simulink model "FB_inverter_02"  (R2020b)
settings: Solver=ode23t  StartTime=0.0  StopTime=0.001  MaxStep=1e-5  RelTol=1e-5
libraries: powerlib x7, simulink x2

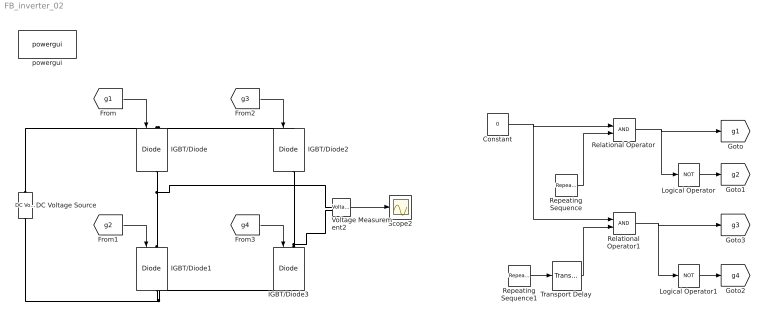
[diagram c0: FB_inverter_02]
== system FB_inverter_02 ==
  Constant : Constant  Value=0
  DC Voltage Source : powerlib/Electrical Sources/DC Voltage Source  Amplitude=400  Measurements=None
  IGBT/Diode{,1..3} (4 alike) : powerlib/Power Electronics/IGBT//Diode  Ron=1e-3  Rs=1e5  Cs=inf  Measurements=on
  Logical Operator : Logic  Operator=NOT  AllPortsSameDT=off  OutDataTypeStr=boolean
  Logical Operator1 : Logic  Operator=NOT  AllPortsSameDT=off  OutDataTypeStr=boolean
  Relational Operator : RelationalOperator  OutDataTypeStr=boolean  RndMeth=Simplest
  Relational Operator1 : RelationalOperator  OutDataTypeStr=boolean  RndMeth=Simplest
  Repeating Sequence : simulink/Sources/Repeating Sequence  rep_seq_t=[0 0.0001 0.0002]  rep_seq_y=[-400 400 -400]
  Repeating Sequence1 : simulink/Sources/Repeating Sequence  rep_seq_t=[0 0.0001 0.0002]  rep_seq_y=[-400 400 -400]
  Scope2 : Scope
  Transport Delay : TransportDelay  DelayTime=0.00001
  Voltage Measurement2 : powerlib/Measurements/Voltage Measurement  PhasorSimulation=off  OutputType=Complex  PSBequivalent=0
  powergui : powerlib/powergui  Priority=1  SimulationMode=Continuous  SampleTime=50e-6  frequency=60  Iterations=50  frequencyindice=0  Pbase=100e6  ErrMax=1e-4  UnitsV=kV  UnitsW=MW  buscounter=0  FunctionMessages=on  echomessages=on  EnableUseOfTLC=off  CurrentSourceSwitches=on  DisableSnubberDevices=on  DisableRonSwitches=on  DisableVfSwitches=on  DisplayEquations=off  AutomaticDiscreteSolvers=off  SolverType=Tustin/Backward Euler (TBE)  Interpol=off  ExternalGateDelay=off  methode=off  Ts=100  x0status=blocks  SPID=on  SwTol=0  HookPort=off  NonlinearTolerance=1e-4  nMaxIteration=100  ContinueOnMaxIteration=off  RestoreLinks=warning  ResistiveCurrentMeasurement=off  Frange=[0:2:500]  Ylog=off  Xlog=on  ShowGrid=off  save=off  variable=ZData  structure=0  ZoomFFT=off  StartTime=0.0  cycles=1  DisplayStyle=1  fundamental=60  FreqAxis=off  MaxFrequency=1000  frequencyindicesteady=1  RmsSteady=1  display=off
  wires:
  [g4] -> IGBT/Diode3/1
  [g2] -> IGBT/Diode1/1
  [g1] -> IGBT/Diode/1
  [g3] -> IGBT/Diode2/1
  Repeating Sequence/1 -> Relational Operator/2
  Constant/1 -> Relational Operator1/1, Relational Operator/1
  Relational Operator/1 -> Logical Operator/1, [g1]
  Logical Operator/1 -> [g2]
  Voltage Measurement2/1 -> Scope2/1
  Repeating Sequence1/1 -> Transport Delay/1
  Relational Operator1/1 -> Logical Operator1/1, [g3]
  Logical Operator1/1 -> [g4]
  Transport Delay/1 -> Relational Operator1/2
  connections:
  IGBT/Diode1/LConn1 -- Voltage Measurement2/LConn1 -- IGBT/Diode/RConn1
  DC Voltage Source/RConn1 -- IGBT/Diode2/LConn1 -- IGBT/Diode/LConn1
  IGBT/Diode1/RConn1 -- DC Voltage Source/LConn1 -- IGBT/Diode3/RConn1
  IGBT/Diode3/LConn1 -- Voltage Measurement2/LConn2 -- IGBT/Diode2/RConn1
